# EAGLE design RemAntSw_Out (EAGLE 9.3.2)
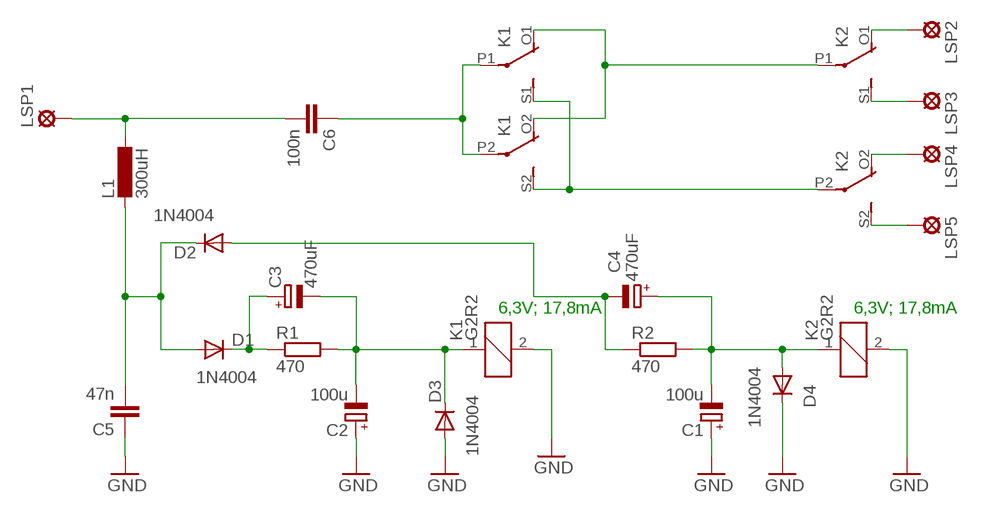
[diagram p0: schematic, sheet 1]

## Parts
C1  100u  CPOL-EUE5-10.5  [E5-10,5]
C2  100u  CPOL-EUE5-10.5  [E5-10,5]
C3  470uF  CPOL-EUE7.5-16  [E7,5-16]
C4  470uF  CPOL-EUE7.5-16  [E7,5-16]
C5  47n  C-EU050-055X075  [C050-055X075]
C6  100n  C-EU050-055X075  [C050-055X075]
D1  1N4004  [DO41-10]
D2  1N4004  [DO41-10]
D3  1N4004  [DO41-10]
D4  1N4004  [DO41-10]
K1  G2R2  [G2R2]
K2  G2R2  [G2R2]
L1  300uH  L-EU6000-XXX-RC  [6000-XXXX-RC]
LSP1  SE14  [SE14]
LSP2  SE14  [SE14]
LSP3  SE14  [SE14]
LSP4  SE14  [SE14]
LSP5  SE14  [SE14]
R1  470  R-EU_0204/5  [0204/5]
R2  470  R-EU_0204/5  [0204/5]

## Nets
GND: C1.+ C2.+ C5.1 D3.A D4.C K1.2 K2.2
N$3: C3.+ D1.C R1.1
N$4: C2.- C3.- D3.C K1.1 R1.2
N$7: K2.O1(2:O) LSP2.MP
N$8: C5.2 D1.A D2.C L1.2
N$9: C4.- D2.A R2.1
N$10: C1.- C4.+ D4.A K2.1 R2.2
N$11: K2.S1(2:S) LSP3.MP
N$12: C6.1 K1.P1(2:P) K1.P2(3:P)
N$13: C6.2 L1.1 LSP1.MP
N$14: K1.O1(2:O) K1.O2(3:O) K2.P1(2:P)
N$15: K1.S1(2:S) K1.S2(3:S) K2.P2(3:P)
N$16: K2.O2(3:O) LSP4.MP
N$17: K2.S2(3:S) LSP5.MP

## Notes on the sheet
- 6,3V; 17,8mA | 6,3V; 17,8mA

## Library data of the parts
C1-C4 = rcl:CPOL-EU: POLARIZED CAPACITOR, European symbol
C5 C6 = rcl:C-EU: CAPACITOR, European symbol
D1-D4 = diode:1N4004: DIODE
K1 K2 = relay:G2R2: RELAY 2 x switch, Omron; MF: OMRON COMPONENTS USA; MPN: G2R-2-DC6; OC_FARNELL: unknown; OC_NEWARK: 89C5317
L1 = rcl:L-EU: INDUCTOR, European symbol
LSP1-LSP5 = solpad:SE14: SOLDER PAD
R1 R2 = rcl:R-EU_: RESISTOR, European symbol

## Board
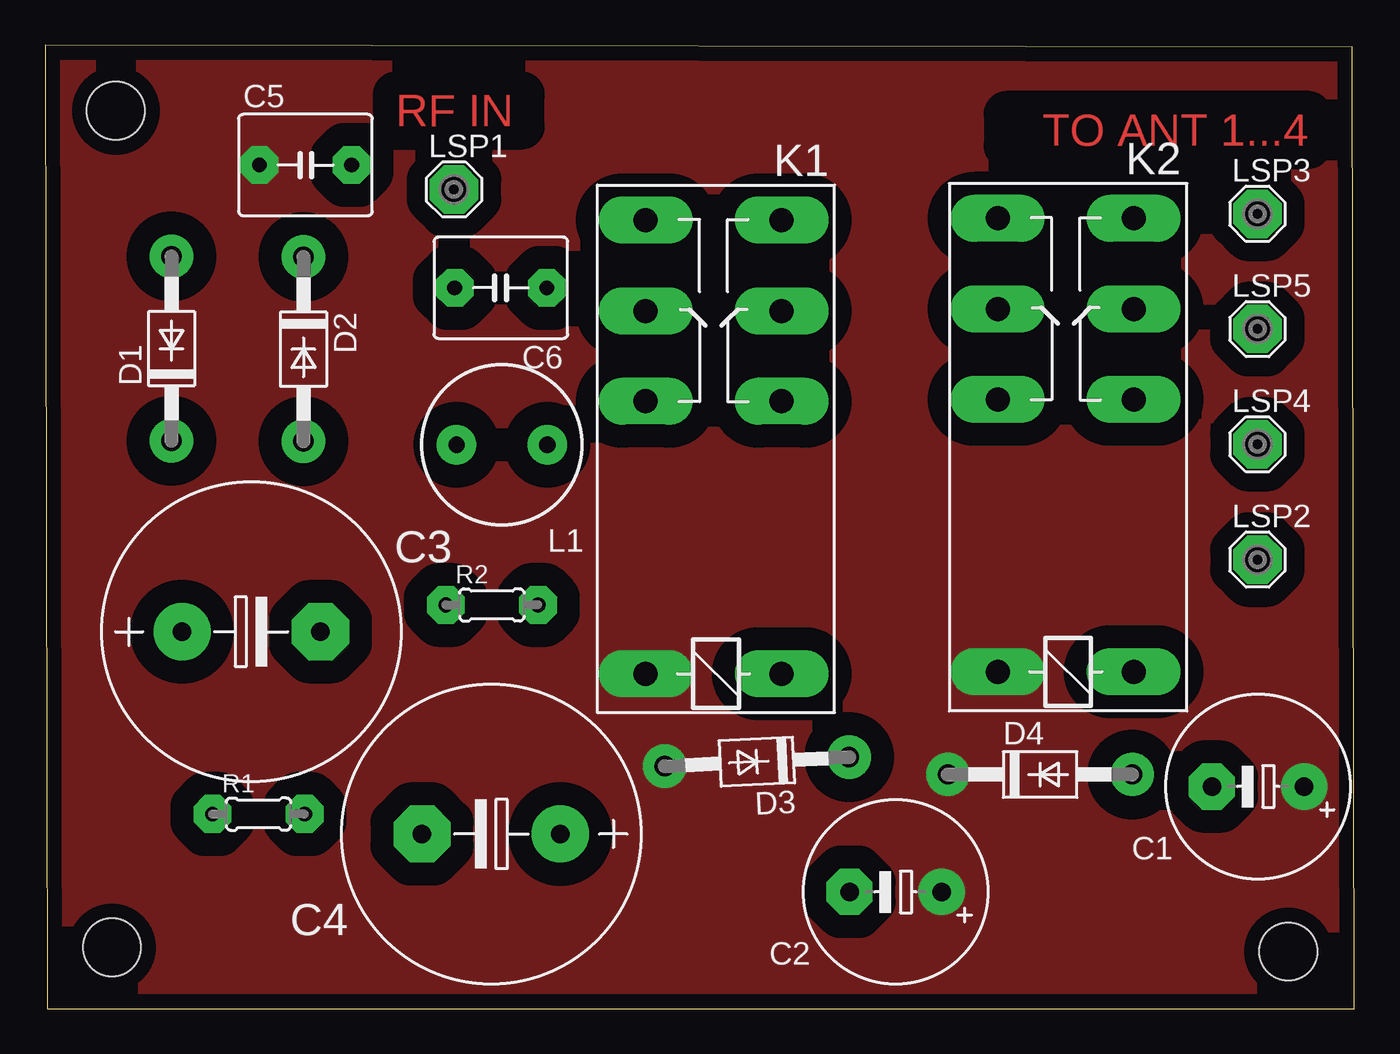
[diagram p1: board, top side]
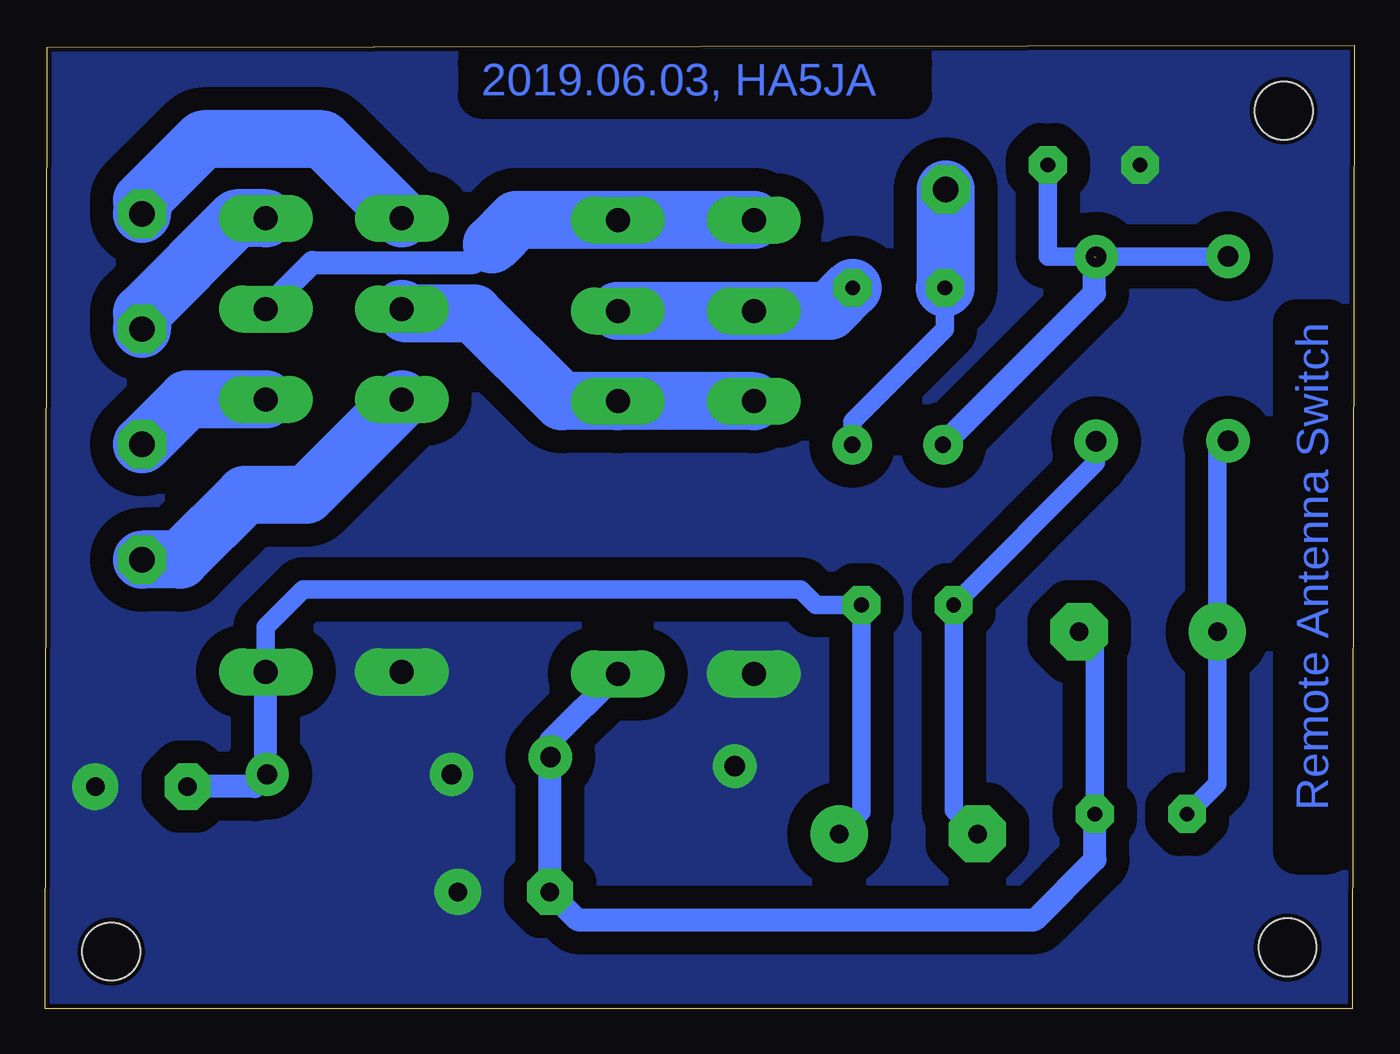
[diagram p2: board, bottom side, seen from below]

Size 72.1 x 53.07 mm. Coordinates in mm from the lower left corner, seen from the top.
Outline: 0.1,0 72.1,0 72,52.97 0,53.07 0.1,0
Copper layers (1*16): Top 0.035mm / dielectric 1.5mm / Bottom 0.035mm
Design rules "default *": minimum track width 10mil, minimum drill 24mil, track to track 50mil, track to pad 35mil, pad to pad 8mil, via to via 8mil, smd to smd 8mil, copper to edge 10mil, drill to drill 8mil, minimum pad ring 25mil, minimum via ring 25mil, stop-mask expansion 4mil, vias tented up to drill 0mil, thermal gap 0mil
Holes 3.2 mm at 3.88,49.47 3.67,3.37 68.47,3.14

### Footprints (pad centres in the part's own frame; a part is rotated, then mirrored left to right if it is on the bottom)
E5-10,5 = drill 1.016 pad 2.54: + -2.54,0 | drill 1.016 pad 2.54 octagon: - 2.54,0
E7,5-16 = drill 1.016 pad 3.15: + -3.81,0 | drill 1.016 pad 3.15 octagon: - 3.81,0
C050-055X075 = drill 0.813 octagon: 1 -2.54,0; 2 2.54,0
DO41-10 = drill 1.118: A 5.08,0; C -5.08,0
G2R2 = drill 1.321 long: 1 -2.54,-3.683; 2 -2.54,3.81; O1 12.471,3.81; O2 12.471,-3.683; P1 17.45,3.81; P2 17.45,-3.683; S1 22.454,3.81; S2 22.454,-3.683
6000-XXXX-RC = drill 0.9 pad 1.422: 1 -2.5,0; 2 2.5,0
SE14 = drill 1.397 pad 2.54 octagon: MP 0,0
0204/5 = drill 0.813 octagon: 1 -2.54,0; 2 2.54,0

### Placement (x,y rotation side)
C1  66.81,12.23 180 top
C2  46.84,6.43 180 top
C3  11.34,20.76 0 top
C4  24.56,9.62 180 top
C5  14.33,46.48 0 top
C6  25.09,39.71 180 top
D1  6.95,36.36 90 top
D2  14.22,36.33 270 top
D3  39.2,13.6 182.8 top
D4  54.8,12.9 0 top
K1  36.88,20.99 90 top
K2  56.28,21.09 90 top
L1  25.15,31.07 180 top
LSP1  22.51,45.13 0 top
LSP2  66.77,24.74 0 top
LSP3  66.77,43.79 0 top
LSP4  66.77,31.09 0 top
LSP5  66.77,37.44 0 top
R1  11.74,10.72 0 top
R2  24.6,22.24 0 top

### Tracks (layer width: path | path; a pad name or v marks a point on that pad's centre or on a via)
GND
  pour Top (isolate 0.813): 0.1,0 72.1,0 72.1,52.98 0.1,52.98
  pour Bottom: 71.9,53.2 71.9,0 0.4,0 0.4,53.2
N$3
  Bottom 1.016: D1.C 7.53,30.7 C3.+ 7.53,12.39 R1.1
N$4
  Bottom 1.016: C3.- 14.28,19.89 R1.2 14.38,10.72
  Bottom 1.27: R1.2 14.28,8.22 17.6,4.9 42.77,4.9 C2.- 44.3,13.82 D3.C 44.27,14.74 K1.1
N$7
  Bottom 3.2: K2.O1 57.73,28.3 61.1,28.3 64.66,24.74 LSP2.MP
N$8  (1 unrouted)
  Top 1.016: 22.8,31.22 L1.2
  Bottom 1.016: D1.A 14.3,41.44 16.87,41.44 C5.2
  Bottom 1.27: L1.2 14.3,39.42 14.3,41.44
N$9
  Bottom 1.016: C4.- 22.06,10.93 R2.1 14.22,30.08 D2.A
N$10
  Bottom 1.016: C4.+ 27.14,10.85 R2.2 29.64,22.24 30.5,23.1 57.9,23.1 59.96,21.04 K2.1 | C1.- 64.36,12.32
  Bottom 1.27: K2.1 59.96,12.98 D4.A 60.55,12.23 C1.-
N$11
  Bottom 3.2: K2.S1 56.83,47.9 63.4,47.9 66.77,44.53 LSP3.MP
N$12
  Bottom 3.2: C6.1 28.9,38.44 K1.P1 K1.P2
N$13
  Bottom 1.016: C6.2 22.55,37.45 27.65,32.35 L1.1
  Bottom 3.2: LSP1.MP 22.51,39.75 C6.2
N$14
  Bottom 3.2: K1.O1 K1.O2 43.66,33.46 48.5,38.3 52.23,38.3 K2.P1
N$15
  Bottom 1.27: K2.P2 57.4,41.1 48.5,41.1 47.5,42.1
  Bottom 3.2: K1.S1 K1.S2 46.16,43.44 47.5,42.1
N$16
  Bottom 3.2: K2.O2 64.3,33.56 LSP4.MP
N$17
  Bottom 3.2: K2.S2 61.56,43.54 66.77,38.33 LSP5.MP

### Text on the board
Top: RF IN | TO ANT 1...4
Bottom: 2019.06.03, HA5JA | Remote Antenna Switch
